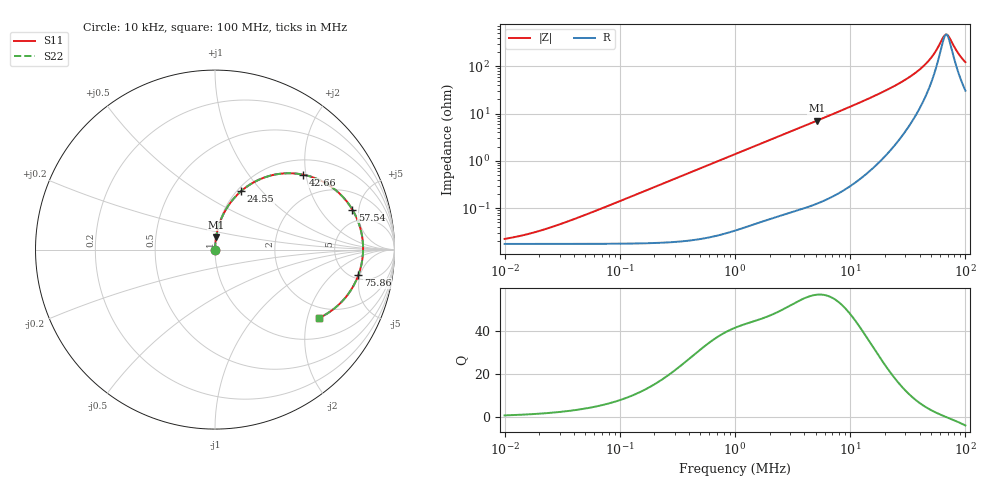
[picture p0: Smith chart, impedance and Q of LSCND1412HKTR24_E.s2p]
! LSCND1412HKTR24_E  S-PARAMETER MODEL  ( Standard Model )
! Model Generated by TAIYO YUDEN Corporation (http://www.ty-top.com)
! Version 1.0
! TAIYO YUDEN Control No. 220401
! Copyright(c) 2022 TAIYO YUDEN CO.,LTD. All Rights Reserved.
! Product Description (link to TY-COMPAS)
! https://ds.yuden.co.jp/TYCOMPAS/or/detail?pn=LSCND1412HKTR24ME&u=M
! Products Name : Inductors
! Characteristics :
!  Inductance : 0.24 [uH] , SRF(min) : - [Hz] , DC Resistance(max) : 22 [mOhm]
!  Rated Current : Saturation  6.5 [A] (dL = 30 [%]), Temp Rise  4.4 [A] (dT = 40 [degC])
!  Case Size : 1.4 x 1.2 / 0.055 x 0.047 [mm/inch] , Thickness : 0.8 / 0.031 [mm/inch]
!  (Conditions: Temperature = 25 [degC] , DC Bias Current = 0 [A])
! External Node Assignments :
!  1  o---GGG---o  2
! GND o---------o GND
! Frequency Range : 10kHz  -  100MHz  [ 402 STEP ]
# MHz S RI R 50
! Freq[MHz].  S11 Real  S11 Imag  S21 Real  S21 Imag  S12 Real  S12 Imag  S22 Real  S22 Imag
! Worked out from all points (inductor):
!   401 points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, 10 kHz to 100 MHz, reference 50 ohm
!   read as one part in series: L = 222 nH near 38.02 kHz
!   highest Q = 56.9 at 5.129 MHz (marker M1), where L = 219 nH
!   self-resonance near 68.28 MHz
!   S11 on the Smith chart (normalised r, x): 10 kHz: 1.00, +0.00; 24.55 MHz: 1.04, +0.78; 42.66 MHz: 1.35, +1.92; 57.54 MHz: 3.49, +4.26; 75.86 MHz: 5.68, -4.69; 100 MHz: 1.61, -2.36
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0.01  0.000175 0.000139  0.9998 -0.000139  0.9998 -0.000139  0.000175 0.000139
0.019953  0.000175 0.000278  0.9998 -0.000278  0.9998 -0.000278  0.000175 0.000278
0.046774  0.000176 0.000652  0.9998 -0.000652  0.9998 -0.000652  0.000176 0.000652
0.218776  0.000194 0.00305  0.9998 -0.00305  0.9998 -0.00305  0.000194 0.00305
1  0.000526 0.0139  0.9995 -0.0139  0.9995 -0.0139  0.000526 0.0139
4.677351  0.00523 0.0638  0.9948 -0.0638  0.9948 -0.0638  0.00523 0.0638
5.128614  0.00616 0.0699  0.9938 -0.0699  0.9938 -0.0699  0.00616 0.0699
11.22019  0.0275 0.1527  0.9725 -0.1527  0.9725 -0.1527  0.0275 0.1527
16.2181  0.0589 0.2202  0.9411 -0.2202  0.9411 -0.2202  0.0589 0.2202
21.87762  0.1126 0.2936  0.8874 -0.2936  0.8874 -0.2936  0.1126 0.2936
24.54709  0.1455 0.3257  0.8545 -0.3257  0.8545 -0.3257  0.1455 0.3257
32.35937  0.2713 0.4004  0.7287 -0.4004  0.7287 -0.4004  0.2713 0.4004
42.65795  0.49 0.4178  0.51 -0.4178  0.51 -0.4178  0.49 0.4178
50.11872  0.6487 0.3495  0.3513 -0.3495  0.3513 -0.3495  0.6487 0.3495
57.54399  0.7657 0.2225  0.2343 -0.2225  0.2343 -0.2225  0.7657 0.2225
64.56542  0.8193 0.0767  0.1807 -0.0767  0.1807 -0.0767  0.8193 0.0767
67.6083  0.8252 0.0135  0.1748 -0.0135  0.1748 -0.0135  0.8252 0.0135
70.79458  0.8217 -0.0498  0.1783 0.0498  0.1783 0.0498  0.8217 -0.0498
75.85776  0.7994 -0.1408  0.2006 0.1408  0.2006 0.1408  0.7994 -0.1408
87.09636  0.7063 -0.2903  0.2937 0.2903  0.2937 0.2903  0.7063 -0.2903
95.49926  0.6229 -0.3576  0.3771 0.3576  0.3771 0.3576  0.6229 -0.3576
100  0.579 -0.3812  0.421 0.3812  0.421 0.3812  0.579 -0.3812
